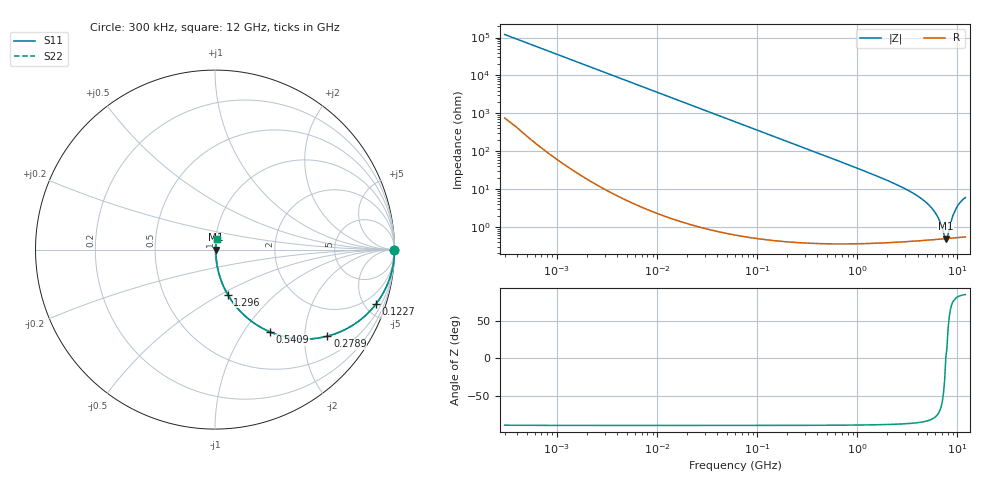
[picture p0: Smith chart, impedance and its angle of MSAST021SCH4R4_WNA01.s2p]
! MSAST021SCH4R4_WNA01  S-PARAMETER MODEL  ( General Type )
! Model Generated by TAIYO YUDEN Corporation (http://www.ty-top.com)
! Version 2.0
! TAIYO YUDEN Control No. 181101
! Copyright(c) 2015 TAIYO YUDEN CO.,LTD. All Rights Reserved.
! Product Description (link to TY-COMPAS)
! https://ds.yuden.co.jp/TYCOMPAS/or/detail?pn=MSAST021SCH4R4BWNA01&u=M
! Products Name : Multilayer Ceramic Capacitors
! Characteristics :
!  Capacitance : 4.4 pF , Rated Voltage : 25V , TCC : CH / C0H
!  Case Size : 0.25 x 0.125 / 0.0098 x 0.0049 [mm/inch] , Thickness : 0.125 / 0.0049 [mm/inch]
!  (Conditions: Temperature = 25 degC , DC Bias Current/Voltage = 0A / 0V)
! External Node Assignments :
!  1  o---| |---o  2
! GND o---------o GND
! Frequency Range : 0.3MHz  -  12000MHz  [ 401 STEP ]
# MHz S RI R 50
! Freq[MHz].  S11 Real  S11 Imag  S21 Real  S21 Imag  S12 Real  S12 Imag  S22 Real  S22 Imag
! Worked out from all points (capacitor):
!   401 points, 300 kHz to 12 GHz, reference 50 ohm
!   read as one part in series: C = 4.4 pF near 316.3 kHz
!   lowest |Z| = 492 mohm at 7.649 GHz (marker M1)
!   series resonance near 7.65 GHz, so ESL is about 98 pH
!   S11 on the Smith chart (normalised r, x): 300 kHz: open; 122.7 MHz: 1.01, -5.90; 278.9 MHz: 1.01, -2.59; 540.9 MHz: 1.01, -1.33; 1.296 GHz: 1.01, -0.54; 12 GHz: 1.01, +0.12
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0.3  1 -0.000829  5.86e-06 0.000829  5.86e-06 0.000829  1 -0.000829
1.769972  1 -0.00489  2.93e-05 0.00489  2.93e-05 0.00489  1 -0.00489
10.44266  0.9991 -0.0288  0.000851 0.0288  0.000851 0.0288  0.9991 -0.0288
60  0.9731 -0.1614  0.0269 0.1614  0.0269 0.1614  0.9731 -0.1614
122.6847  0.8964 -0.304  0.1036 0.304  0.1036 0.304  0.8964 -0.304
278.9009  0.6262 -0.4823  0.3738 0.4823  0.3738 0.4823  0.6262 -0.4823
353.9943  0.5097 -0.4981  0.4903 0.4981  0.4903 0.4981  0.5097 -0.4981
540.8523  0.3079 -0.4589  0.6921 0.4589  0.6921 0.4589  0.3079 -0.4589
826.3444  0.1597 -0.3622  0.8403 0.3622  0.8403 0.3622  0.1597 -0.3622
1296.429  0.0714 -0.2508  0.9286 0.2508  0.9286 0.2508  0.0714 -0.2508
2088.533  0.0286 -0.1551  0.9714 0.1551  0.9714 0.1551  0.0286 -0.1551
3642.919  0.01 -0.0758  0.99 0.0758  0.99 0.0758  0.01 -0.0758
5140.631  0.00597 -0.0383  0.994 0.0383  0.994 0.0383  0.00597 -0.0383
6188.031  0.00508 -0.0202  0.9949 0.0202  0.9949 0.0202  0.00508 -0.0202
6699.894  0.00491 -0.0126  0.9951 0.0126  0.9951 0.0126  0.00491 -0.0126
7254.098  0.00486 -0.00514  0.9951 0.00514  0.9951 0.00514  0.00486 -0.00514
7648.807  0.0049 -5.96e-06  0.9951 5.96e-06  0.9951 5.96e-06  0.0049 -5.96e-06
8064.993  0.00497 0.00407  0.995 -0.00407  0.995 -0.00407  0.00497 0.00407
8966.534  0.00542 0.0186  0.9946 -0.0186  0.9946 -0.0186  0.00542 0.0186
9708.23  0.00608 0.0302  0.9939 -0.0302  0.9939 -0.0302  0.00608 0.0302
10793.46  0.0074 0.0457  0.9926 -0.0457  0.9926 -0.0457  0.0074 0.0457
12000  0.00894 0.0589  0.9911 -0.0589  0.9911 -0.0589  0.00894 0.0589
